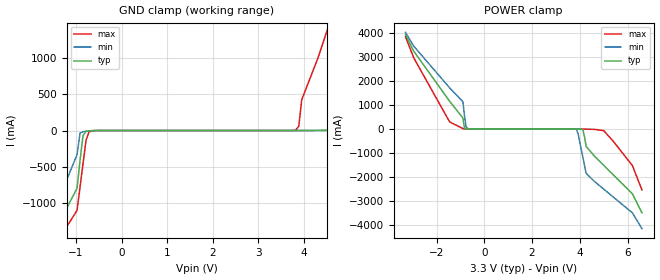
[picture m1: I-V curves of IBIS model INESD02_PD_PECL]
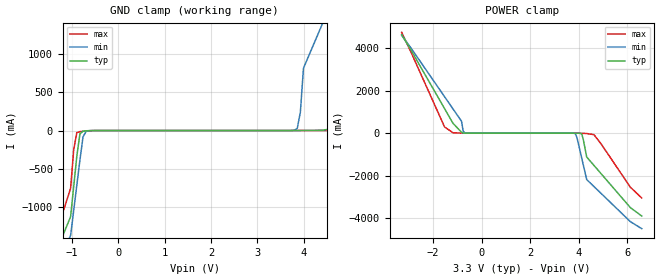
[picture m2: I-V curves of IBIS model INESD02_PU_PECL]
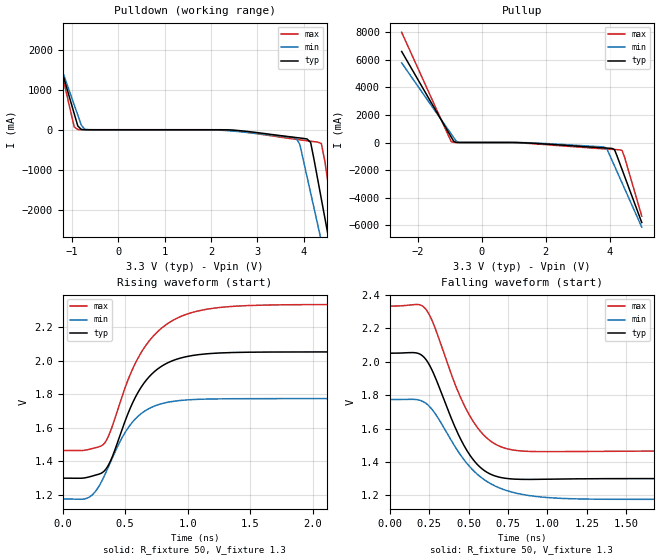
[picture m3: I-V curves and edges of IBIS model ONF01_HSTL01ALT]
|   This file is an IBIS representation of the   |
|   Integrated Devices Technology, Inc.   |
|   ICS85356I   |
|   Dual LVPECL/ECL  Clock Multiplexer   |
[IBIS Ver]   4.1
[File name]   85356i_3v3.ibs
[File Rev]   1.0
[Date]   19 Mar 2009 | Last modified
|   Mar 24 2003 | Generated
[Source]   Originated at Integrated Devices Technology, Inc.
[Disclaimer]
IDT hereby grants the user of this IBIS model a non-exclusive,
nontransferable license to use this IBIS model under the following terms.
Before using this IBIS model, the user should read this license.
If the user does not accept these terms,  the IBIS model should be
returned to IDT within 30 days.
   The user is granted this license only to use the IBIS model and
is not granted rights to sell, load, rent, lease or license the IBIS
model in whole or in part, or in modified form to anyone other than
user. User may modify the IBIS model to suit its specific
applications but rights to derivative works and such modifications
shall belong to IDT.
   This IBIS model is provided on an "AS IS" basis and IDT makes
absolutely no warranty with respect to the information contained
herein. IDT DISCLAIMS AND CUSTOMER WAIVES ALL WARRANTIES, EXPRESS
OR IMPLIED, INCLUDING WARRANTIES OF MERCHANTABILITY OR FITNESS FOR
A PARTICULAR PURPOSE. The entire risk as to quality and performance
is with the Customer. ACCORDINGLY, IN NO EVENT SHALL THE COMPANY BE
LIABLE FOR ANY DAMAGES, WHETHER IN CONTRACT OR TORT,INCLUDING ANY
LOST PROFITS OR OTHER INCIDENTAL, CONSEQUENTIAL, EXEMPLARY, OR
PUNITIVE DAMAGES ARISING OUT OF THE USE OR APPLICATION OF THE IBIS
model provided in this package. Further, IDT reserves the right to
make changes without notice to any product herein to improve
reliability, function, or design. IDT does not convey any license
under patent rights or any other intellectual property rights,
including those of third parties.
   IDT is not obligated to provide maintenance or support
for the licensed IBIS model.
[Copyright]   Copyright 2003 by Integrated Devices Technology, Inc.
[Component]   ICS85356AMI
[Manufacturer] Integrated Devices Technology, Inc.
[Package]
|SOIC 20 Lead
|   typ   min   max
R_pkg   57.15m   45.4m   68.9m
L_pkg   4.051nH   2.187nH   5.914nH
C_pkg   0.796pF   0.419pF   1.173pF
[Pin]  signal_name   model_name   R_pin   L_pin   C_pin
1   CLK0A   INESD02_PD_PECL   68.90m   5.914n   1.173p
2   nCLK0A   INESD02_PU_PECL   63.02m   4.983n   0.985p
3   nc   nc   57.15m   4.051n   0.796p
4   CLK0B   INESD02_PD_PECL   51.25m   3.119n   0.608p
5   nCLK0B   INESD02_PU_PECL   45.40m   2.187n   0.419p
6   CLK1A   INESD02_PD_PECL   45.40m   2.187n   0.419p
7   nCLK1A   INESD02_PU_PECL   51.25m   3.119n   0.608p
8   nc   nc   57.15m   4.051n   0.796p
9   CLK1B   INESD02_PD_PECL   63.02m   4.983n   0.985p
10   nCLK1B   INESD02_PU_PECL   68.90m   5.914n   1.173p
11   VEE   GND   68.90m   5.914n   1.173p
12   nQ1   ONF01_HSTL01ALT   63.02m   4.983n   0.985p
13   Q1   ONF01_HSTL01ALT   57.15m   4.051n   0.796p
14   VCC   POWER   51.25m   3.119n   0.608p
15   SEL1   INESD01_PU_PECL   45.40m   2.187n   0.419p
16   COM_SEL   INESD01_PD_PECL   45.40m   2.187n   0.419p
17   SEL0   INESD01_PU_PECL   51.25m   3.119n   0.608p
18   nQ0   ONF01_HSTL01ALT   57.15m   4.051n   0.796p
19   Q0   ONF01_HSTL01ALT   63.02m   4.983n   0.985p
20   VCC   POWER   68.90m   5.914n   1.173p
[Diff Pin]  inv_pin  vdiff tdelay_typ tdelay_min  tdelay_max
|Input
1   2   .15  0  0  0
4   5   .15  0  0  0
6   7   .15  0  0  0
9   10   .15  0  0  0
|Output
13   12   NA   0  0  0
19   18   NA   0  0  0
[Component]   ICS85356AGI
[Manufacturer] Integrated Devices Technology, Inc.
[Package]
|TSSOP 20 Lead
|   typ   min   max
R_pkg   51.85m   41.1m   62.6m
L_pkg   1.568nH   0.734nH   2.401nH
C_pkg   0.221pF   0.068pF   0.373pF
[Pin]  signal_name   model_name   R_pin   L_pin   C_pin
1   CLK0A   INESD02_PD_PECL   62.6m   2.401n   0.373p
2   nCLK0A   INESD02_PU_PECL   57.23m   1.985n   0.297p
|3   nc   nc   51.85m   1.568n   0.221p
4   CLK0B   INESD02_PD_PECL   46.78m   1.151n   0.145p
5   nCLK0B   INESD02_PU_PECL   41.1m   0.734n   0.068p
6   CLK1A   INESD02_PD_PECL   41.1m   0.734n   0.068p
7   nCLK1A   INESD02_PU_PECL   46.78m   1.151n   0.145p
|8   nc   nc   51.85m   1.568n   0.221p
9   CLK1B   INESD02_PD_PECL   57.23m   1.985n   0.297p
10   nCLK1B   INESD02_PU_PECL   62.6m   2.401n   0.373p
11   VEE   GND   62.6m   2.401n   0.373p
12   nQ1   ONF01_HSTL01ALT   57.23m   1.985n   0.297p
13   Q1   ONF01_HSTL01ALT   51.85m   1.568n   0.221p
14   VCC   POWER   46.78m   1.151n   0.145p
15   SEL1   INESD01_PU_PECL   41.1m   0.734n   0.068p
16   COM_SEL   INESD01_PD_PECL   41.1m   0.734n   0.068p
17   SEL0   INESD01_PU_PECL   46.78m   1.151n   0.145p
18   nQ0   ONF01_HSTL01ALT   51.85m   1.568n   0.221p
19   Q0   ONF01_HSTL01ALT   57.23m   1.985n   0.297p
20   VCC   POWER   62.6m   2.401n   0.373p
[Diff Pin]  inv_pin  vdiff tdelay_typ tdelay_min  tdelay_max
|Input
1   2   .15  0  0  0
4   5   .15  0  0  0
6   7   .15  0  0  0
9   10   .15  0  0  0
|Output
13   12   NA   0  0  0
19   18   NA   0  0  0
| Models and submodels in the file (5): INESD02_PD_PECL (Input), INESD02_PU_PECL (Input), ONF01_HSTL01ALT (Output_ECL), INESD01_PU_PECL (Input), INESD01_PD_PECL (Input)
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[Model]   INESD02_PD_PECL
Model_type  Input
Polarity   Non-Inverting
Vinl = 0.8V
Vinh = 2.0V
|   typ   min   max
C_comp   2pF   1.5pF   2.5pF
|   typ   min   max
[Voltage range]  3.3V   3.15V   3.45V
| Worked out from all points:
|   GND clamp passes 1 mA (typ) near -0.59 V on its own axis
|   POWER clamp passes 1 mA (typ) near -0.70 V on its own axis
[GND_clamp]
-3.3V     -3.894A    -4.294A    -3.674A
-1.6V     -1.569A    -1.322A    -1.74A
-974.8mV  -794.1mA   -331.5mA   -1.096A
-843.4mV  -68.33mA   -15.34mA   -452.9mA
-646.5mV  -1.912mA   -4.151mA   -2.665mA
3.818V    89.38uA    70.49uA    7.198mA
3.95V     342.2uA    75.94uA    423.8mA
4.6V      7.437mA    165.5uA    1.553A
4.9V      78.32mA    440.9uA    2.118A
5.5V      1.293A     2.769mA    3.249A
6.25V     2.651A     112.4mA    4.38A
6.6V      3.331A     896.1mA    4.946A
[POWER_clamp]
-3.3V     3.923A     4.017A     3.838A
-2.95V    3.23A      3.44A      2.951A
-1.45V    1.149A     1.709A     289.6mA
-896.9mV  456.5mA    1.133A     15.4mA
-762.9mV  4.223mA    91.07mA    1.486mA
-695.9mV  792.2uA    10.73mA    555.6uA
3.861V    -556.7uA   -26.14mA   -39.45uA
4.129V    -41.85mA   -1.19A     -4.904mA
4.263V    -724.2mA   -1.847A    -12.04mA
5V        -1.514A    -2.505A    -71.38mA
6.2V      -2.701A    -3.492A    -1.525A
6.6V      -3.492A    -4.151A    -2.536A
[Model]   INESD02_PU_PECL
Model_type  Input
Polarity   Non-Inverting
Vinl = 0.8V
Vinh = 2.0V
|   typ   min   max
C_comp   2pF   1.5pF   2.5pF
|   typ   min   max
[Voltage range]  3.3V   3.15V   3.45V
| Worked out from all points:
|   GND clamp passes 1 mA (typ) near -0.59 V on its own axis
|   POWER clamp passes 1 mA (typ) near -0.70 V on its own axis
[GND_clamp]
|Voltage   I(typ)   I(min)   I(max)
-3.3V     -3.894A    -3.674A    -4.294A
-1.3V     -1.521A    -1.7A      -1.261A
-1.031V   -1.125A    -1.372A    -755.3mA
-896.9mV  -335.4mA   -714.7mA   -27.07mA
-695.9mV  -3.401mA   -10.69mA   -6.477mA
3.794V    17.99uA    3.319mA    6.081uA
3.928V    181.1uA    239mA      10.12uA
3.995V    711.6uA    813.7mA    20.78uA
4.8V      40.44mA    1.967A     268.6uA
5.6V      1.139A     3.12A      2.243mA
6.3V      2.525A     4.275A     64.01mA
6.6V      3.219A     4.852A     752.7mA
[POWER_clamp]
|Voltage   I(typ)   I(min)   I(max)
-3.3V     4.617A     4.594A     4.726A
-1.53V    1.149A     1.709A     289.6mA
-1.18V    456.4mA    1.132A     15.33mA
-829.9mV  42.02mA    556.1mA    3.39mA
-762.9mV  4.159mA    91mA       1.422mA
-695.9mV  727.9uA    10.66mA    491.6uA
3.861V    -620.9uA   -26.2mA    -103.4uA
4.129V    -41.91mA   -1.19A     -4.968mA
4.33V     -1.119A    -2.176A    -17.93mA
4.63V     -1.515A    -2.505A    -71.45mA
6.13V     -3.492A    -4.151A    -2.536A
6.6V      -3.888A    -4.48A     -3.041A
[Model]   ONF01_HSTL01ALT
Model_type  Output_ECL
Polarity   Non-Inverting
Vmeas = 1.5
Rref = 50
Cref = 0
Vref = 1.3
|Variable  typ   min   max
C_comp   2p   1.5p   2.5p
[Voltage Range]   3.3   3.135   3.465
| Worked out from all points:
|   rising waveform, R_fixture 50, V_fixture 1.3: 20-80 % time 280ps typ, 262ps min, 333ps max; typ from 1.3 V to 2.05 V
|   falling waveform, R_fixture 50, V_fixture 1.3: 20-80 % time 210ps typ, 283ps min, 228ps max; typ from 2.05 V to 1.3 V
| Open source, no load
|  Voltage   I(typ)   I(min)   I(max)
[Pullup]
-2.5V     6.581A     5.758A     7.966A
-953.6mV  402.1mA    621.9mA    72.14mA
-876.3mV  95.6mA     366.6mA    5.897mA
-799mV    6.347mA    111.8mA    2.212mA
-721.6mV  951.4uA    9.59mA     751.4uA
1.057V    -2.168mA   -472.7uA   -9.007mA
3.84V     -393.7mA   -335.2mA   -462.5mA
3.918V    -404.3mA   -490.1mA   -473.9mA
4.149V    -514.4mA   -1.696A    -507.3mA
4.381V    -1.931A    -2.903A    -564.7mA
4.459V    -2.413A    -3.305A    -1.021A
5V        -5.786A    -6.12A     -5.32A
[Pulldown]
-2.5V     6.581A     5.758A     7.966A
-1.495V   2.559A     2.415A     2.824A
-1.418V   2.25A      2.158A     2.429A
-953.6mV  402.1mA    621.9mA    72.14mA
-876.3mV  95.6mA     366.6mA    5.897mA
-721.6mV  951.4uA    9.59mA     751.4uA
3.84V     -195.1mA   -215.5mA   -239.9mA
4.149V    -316mA     -1.576A    -286.2mA
4.381V    -1.732A    -2.781A    -344.8mA
4.536V    -2.697A    -3.585A    -1.416A
4.691V    -3.661A    -4.389A    -2.646A
5V        -5.591A    -5.997A    -5.105A
[Ramp]
|   typ   min   max
dV/dt_r   0.601/0.450n   0.479/0.414n   0.695/0.533n
dV/dt_f   0.607/0.317n   0.479/0.450n   0.705/0.343n
R_load =   50.0000
[Rising Waveform]
R_fixture = 50
V_fixture = 1.3   | VCC_typ - 2V
V_fixture_max = 1.465   | VCC_max - 2V
V_fixture_min = 1.135   | VCC_min - 2V
C_fixture = 0.0p
| Time   typ   min   max
0s        1.3V       1.176V     1.465V
207.7ps   1.307V     1.185V     1.471V
331.7ps   1.342V     1.312V     1.506V
390.6ps   1.417V     1.41V      1.597V
492.9ps   1.628V     1.564V     1.826V
632.4ps   1.847V     1.687V     2.053V
775ps     1.958V     1.74V      2.183V
964.1ps   2.019V     1.764V     2.268V
1.463ns   2.049V     1.773V     2.327V
2.998ns   2.051V     1.773V     2.334V
[Falling Waveform]
R_fixture = 50
V_fixture = 1.3   | VCC_typ - 2V
V_fixture_max = 1.465   | VCC_max - 2V
V_fixture_min = 1.135   | VCC_min - 2V
C_fixture = 0.0p
| Time   typ   min   max
0s        2.051V     1.773V     2.334V
167.4ps   2.053V     1.774V     2.343V
229.4ps   2.014V     1.751V     2.315V
282.1ps   1.922V     1.698V     2.216V
427.8ps   1.58V      1.472V     1.834V
505.3ps   1.445V     1.374V     1.68V
610.7ps   1.341V     1.286V     1.548V
728.5ps   1.302V     1.232V     1.483V
1.175ns   1.298V     1.179V     1.462V
2.998ns   1.3V       1.176V     1.465V
